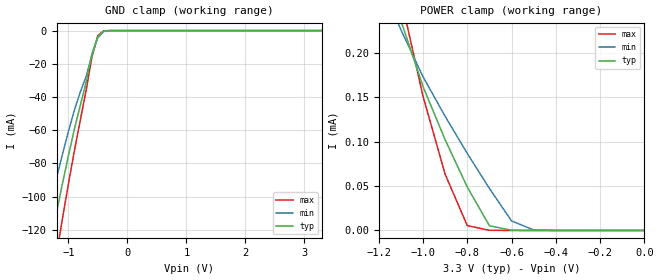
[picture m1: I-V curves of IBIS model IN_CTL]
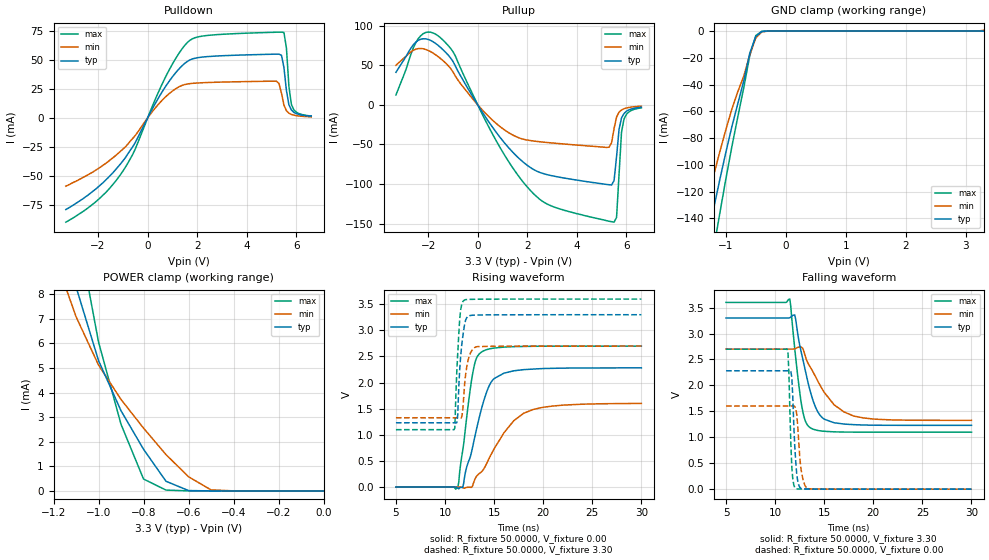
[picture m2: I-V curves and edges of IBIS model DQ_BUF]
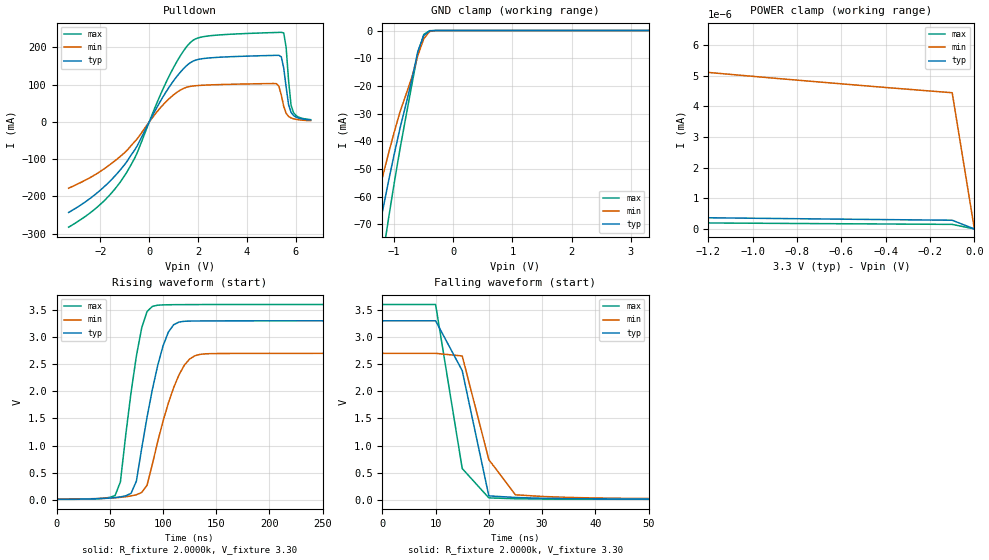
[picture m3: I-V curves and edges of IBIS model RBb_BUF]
| This IBIS file was created by s2ibis3 version 1.1
| North Carolina State University, ERL, 2006
[IBIS ver] 3.2
[File name] s34ml02g2_d_i_33_r2.ibs
[File Rev] 2.0
|   Rev1.0 Initial release with measurement
|   (X8 Legacy/ONFI F32 98799A 41122)
|   Rev2.0 Update 0A for 0V
[Date] 7/23/2014
[Source] Spansion IBIS team
|   Email: dl.ibisteam@spansion.com
[Notes]  Generated IBIS models from SPICE simulations.
|   VIO=3.3V, Temperature Range: Industrial (-40oC to +90oC).
[Disclaimer] THE MODEL LIBRARIES ARE PROVIDED AS IS.
[Copyright] (C) COPYRIGHT 2014
| SPANSION LLC
| ALL RIGHTS RESERVED.
|   Component S34ML02G2 X8 LEGACY/ONFI F32 in VBT067 package
[Component]   S34ML02G2
[Manufacturer]   Spansion
[Package]
| variable   typ   min   max
R_pkg   139.8mOhm   83.414mOhm   221.06mOhm
L_pkg   4.331nH   2.162nH   7.708nH
C_pkg   0.8614pF   0.3971pF   1.325pF
[Pin]   signal_name   model_name   R_pin   L_pin   C_pin
A2   NC   NC
A3   NC   NC
A6   NC   NC
A7   NC   NC
A8   NC   NC
B1   NC   NC
B2   WP   IN_CTL   186.22m   5.30n   1.33p
B3   ALE   IN_CTL   183.76m   5.66n   1.15p
B4   VSS   GND
B5   CE   IN_CTL   193.1m   7.14n   1.17p
B6   WE   IN_CTL   211.06m   6.84n   1.27p
B7   R/B#   RBb_BUF   176.3m   6.17n   1.11p
B8   NC   NC
C1   NC   NC
C2   NC   NC
C3   RE   IN_CTL   185.42m   7.71n   0.81p
C4   CLE   IN_CTL   170.19m   4.4n   1.18p
C5   NC   NC
C6   NC   NC
C7   NC   NC
C8   NC   NC
D2   NC   NC
D3   NC   NC
D4   NC   NC
D5   NC   NC
D6   NC   NC
D7   NC   NC
E2   NC   NC
E3   NC   NC
E4   NC   NC
E5   NC   NC
E6   NC   NC
E7   NC   NC
F2   NC   NC
F3   NC   NC
F4   NC   NC
F5   NC   NC
F6   NC   NC
F7   NC   NC
G2   NC   NC
G3   IO0   DQ_BUF   109.68m   2.85n   0.779p
G4   NC   NC
G5   NC   NC
G6   NC   NC
G7   VCC   POWER
H1   NC   NC
H2   NC   NC
H3   IO1   DQ_BUF   96.013m   2.44n   0.655p
H4   NC   NC
H5   VCC   POWER
H6   IO5   DQ_BUF   105.71m   3.38n   0.558p
H7   IO7   DQ_BUF   110.99m   3.27n   0.735p
H8   NC   NC
J1   NC   NC
J2   VSS   GND
J3   IO2   DQ_BUF   89.696m   2.19n   0.633p
J4   IO3   DQ_BUF   93.132m   2.31n   0.589p
J5   IO4   DQ_BUF   102.28m   3.14n   0.574p
J6   IO6   DQ_BUF   83.414m   2.16n   0.392p
J7   VSS   GND
J8   NC   NC
K1   NC   NC
K2   NC   NC
K3   NC   NC
K6   NC   NC
K7   NC   NC
K8   NC   NC
| Models and submodels in the file (3): IN_CTL (Input), DQ_BUF (I/O), RBb_BUF (Open_drain)
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|   Model IN_CTL
[Model]   IN_CTL
Model_type   Input
Vinl =   1.3180
Vinh =   1.6630
C_comp   6.01pF   5.78pF   8.57pF
[Temperature Range]   25.0000   90.0000   -40.0000
[Voltage Range]   3.3000   2.7000   3.6000
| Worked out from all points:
|   GND clamp passes 1 mA (typ) near -0.42 V on its own axis
|   POWER clamp passes 1 mA (typ) near -1.80 V on its own axis
[GND_clamp]
| voltage   I(typ)   I(min)   I(max)
-3.3V     -563.9mA   -475.7mA   -665.6mA
-1.5V     -164.8mA   -133.7mA   -202.4mA
-1.4V     -145.8mA   -118.2mA   -179.3mA
-1.3V     -127.4mA   -103.2mA   -156.7mA
-1.2V     -109.5mA   -88.65mA   -134.7mA
-1.1V     -92.25mA   -74.51mA   -113.2mA
-900mV    -59.75mA   -48.15mA   -72.81mA
-700mV    -31.42mA   -27.84mA   -36.18mA
-600mV    -14.17mA   -14.52mA   -15.79mA
-500mV    -3.458mA   -4.259mA   -2.945mA
-400mV    -298.7uA   -518.7uA   -127.7uA
3.3V      292.5pA    10.73uA    139.6pA
[POWER_clamp]
| voltage   I(typ)   I(min)   I(max)
-3.3V     27.06A     13.23A     34.66A
-1.1V     236.4uA    226.1uA    262.5uA
-1V       162.2uA    173.2uA    151.3uA
-900mV    102.2uA    128.6uA    63.39uA
-800mV    48.96uA    86.76uA    5.425uA
-700mV    5.388uA    47.41uA    237.2nA
-600mV    176.5nA    10.73uA    6.564nA
-500mV    6.019nA    596nA      279.6pA
0V        0A         0A         0A
|   Model DQ_BUF
[Model]   DQ_BUF
Model_type   I/O
Polarity   Non-Inverting
Enable   Active-High
Vinl =   1.3180
Vinh =   1.6630
Vmeas =   1.65V
C_comp   2.54pF   2.48pF   2.73pF
[Temperature Range]   25.0000   90.0000   -40.0000
[Voltage Range]   3.3000   2.7000   3.6000
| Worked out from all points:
|   slope of the pulldown table from 0 to 0.495 V, typ, clamps not added: 25.6 ohm
|   slope of the pullup table from 0 to 0.495 V, typ, clamps not added: 20.9 ohm
|   GND clamp passes 1 mA (typ) near -0.42 V on its own axis
|   POWER clamp passes 1 mA (typ) near -0.75 V on its own axis
|   rising waveform, R_fixture 50.0000, V_fixture 0.00: 20-80 % time 1.92ns typ, 3.23ns min, 1.14ns max; typ from 0 V to 2.28 V
|   rising waveform, R_fixture 50.0000, V_fixture 3.30: 20-80 % time 465ps typ, 496ps min, 379ps max; typ from 1.23 V to 3.3 V
|   falling waveform, R_fixture 50.0000, V_fixture 3.30: 20-80 % time 1.58ns typ, 2.84ns min, 926ps max; typ from 3.3 V to 1.23 V
|   falling waveform, R_fixture 50.0000, V_fixture 0.00: 20-80 % time 346ps typ, 421ps min, 262ps max; typ from 2.28 V to 0 V
[GND_clamp]
| voltage   I(typ)   I(min)   I(max)
-3.3V     -1.531A    -857.2mA   -2.572A
-1.5V     -199.4mA   -161.9mA   -246.1mA
-1.4V     -176.3mA   -143.2mA   -217.6mA
-1.3V     -153.9mA   -125mA     -189.7mA
-1.2V     -132.2mA   -107.4mA   -162.6mA
-1.1V     -111.1mA   -90.32mA   -136.3mA
-900mV    -71.7mA    -58.5mA    -86.72mA
-700mV    -37.18mA   -33.68mA   -42.32mA
-600mV    -16.53mA   -17.62mA   -18.35mA
-500mV    -4.024mA   -5.179mA   -3.39mA
-400mV    -347uA     -622.1uA   -145.7uA
3.3V      401pA      577.4uA    196.4pA
[POWER_clamp]
| voltage   I(typ)   I(min)   I(max)
-3.3V     28.02A     13.67A     36.43A
-1.2V     12.2mA     9.687mA    16.8mA
-1.1V     8.304mA    7.091mA    10.97mA
-1V       5.304mA    5.122mA    6.06mA
-900mV    3.262mA    3.722mA    2.71mA
-800mV    1.696mA    2.556mA    484.6uA
-700mV    392.2uA    1.477mA    34.23uA
-600mV    15.16uA    577.4uA    1.674uA
-500mV    621.3nA    42.06uA    41.77nA
-400mV    23.44nA    2.247uA    920.4pA
0V        0A         0A         0A
[Pulldown]
| voltage   I(typ)   I(min)   I(max)
-3.3V     -78.9mA    -58.8mA    -89.8mA
-1.1V     -39.8mA    -28.88mA   -49mA
-500mV    -21.23mA   -15.18mA   -26.87mA
900mV     32.53mA    21.5mA     42.55mA
1.8V      50.8mA     29.79mA    68.12mA
5.2V      54.94mA    31.61mA    73.89mA
5.4V      53.96mA    21.3mA     73.98mA
5.5V      43.4mA     11.1mA     73.57mA
5.6V      23.6mA     6.2mA      60.2mA
5.7V      11.3mA     4.1mA      27.2mA
5.8V      6.9mA      3mA        11.6mA
6.6V      1.6mA      900uA      1.8mA
[Pullup]
| voltage   I(typ)   I(min)   I(max)
-3.3V     41mA       49.8mA     12.4mA
-2.4V     81.3mA     70.88mA    83.4mA
-1.7V     77.37mA    63.08mA    89.09mA
-1V       54.74mA    41.53mA    67.09mA
700mV     -32.73mA   -22.28mA   -42.8mA
2.2V      -80.59mA   -45.42mA   -110.5mA
5.3V      -100.8mA   -53.4mA    -146.8mA
5.5V      -95.4mA    -29.8mA    -148mA
5.6V      -65.2mA    -15.4mA    -141.9mA
5.8V      -16.5mA    -6.5mA     -34.4mA
5.9V      -11mA      -4.9mA     -18mA
6.6V      -3.1mA     -1.7mA     -3.9mA
[Ramp]
| variable   typ   min   max
dV/dt_r   2.2818/1.922e-09   1.6009/3.212e-09   2.6978/1.138e-09
dV/dt_f   2.0696/1.584e-09   1.3732/2.799e-09   2.5018/9.242e-10
R_load = 50.0000
[Rising Waveform]
R_fixture = 50.0000
V_fixture = 0.00
| time   V(typ)   V(min)   V(max)
5ns       0V         0V         0V
11.3ns    -21.43mV   33.17uV    -13.34mV
11.8ns    -8.737mV   -10.81mV   695.5mV
12.9ns    842.8mV    76.14mV    2.255V
13.3ns    1.182V     224.4mV    2.504V
13.9ns    1.621V     332.1mV    2.606V
15ns      2.077V     731mV      2.662V
18ns      2.248V     1.411V     2.692V
22ns      2.277V     1.568V     2.697V
30ns      2.282V     1.601V     2.698V
[Rising Waveform]
R_fixture = 50.0000
V_fixture = 3.30
V_fixture_min = 2.70
V_fixture_max = 3.60
| time   V(typ)   V(min)   V(max)
5ns       1.23V      1.327V     1.098V
11ns      1.23V      1.327V     1.126V
11.2ns    1.231V     1.327V     2.214V
11.3ns    1.394V     1.327V     2.572V
11.5ns    2.262V     1.322V     3.228V
11.8ns    2.866V     1.452V     3.546V
12ns      3.122V     1.977V     3.582V
12.5ns    3.283V     2.523V     3.594V
13.2ns    3.294V     2.685V     3.596V
30ns      3.3V       2.7V       3.6V
[Falling Waveform]
R_fixture = 50.0000
V_fixture = 3.30
V_fixture_min = 2.70
V_fixture_max = 3.60
| time   V(typ)   V(min)   V(max)
5ns       3.3V       2.7V       3.6V
11.5ns    3.305V     2.7V       3.664V
12ns      3.357V     2.706V     2.703V
12.7ns    2.606V     2.733V     1.617V
13.1ns    2.264V     2.547V     1.304V
13.7ns    1.805V     2.313V     1.171V
14.3ns    1.507V     2.101V     1.134V
15ns      1.35V      1.866V     1.115V
18ns      1.244V     1.41V      1.1V
30ns      1.23V      1.327V     1.098V
[Falling Waveform]
R_fixture = 50.0000
V_fixture = 0.00
| time   V(typ)   V(min)   V(max)
5ns       2.282V     1.603V     2.698V
11.3ns    2.282V     1.603V     2.671V
11.4ns    2.283V     1.603V     2.243V
11.6ns    2.265V     1.603V     880.5mV
11.7ns    2.158V     1.605V     421.3mV
12.1ns    524.6mV    1.55V      10mV
12.3ns    158.3mV    1.219V     4.58mV
12.6ns    17.13mV    438.4mV    2.749mV
13.3ns    2.691mV    14.67mV    1.287mV
30ns      0V         641.2nV    0V
|   Model RBb_BUF
[Model]   RBb_BUF
Model_type   Open_drain
Polarity   Non-Inverting
Enable   Active-High
Vmeas =   1.65V
Rref =  2.0000k
Vref =  3.3000
C_comp   6.45pF   6.07pF   9.98pF
[Temperature Range]   25.0000   90.0000   -40.0000
[Voltage Range]   3.3000   2.7000   3.6000
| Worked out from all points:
|   slope of the pulldown table from 0 to 0.495 V, typ, clamps not added: 8.28 ohm
|   GND clamp passes 1 mA (typ) near -0.45 V on its own axis
|   POWER clamp passes 1 mA (typ) near -2.01 V on its own axis
|   rising waveform, R_fixture 2.0000k, V_fixture 3.30: 20-80 % time 19.6ns typ, 23.4ns min, 14.9ns max; typ from 0.013 V to 3.3 V
|   falling waveform, R_fixture 2.0000k, V_fixture 3.30: 20-80 % time 5.13ns typ, 5.19ns min, 3.56ns max; typ from 3.3 V to 0.013 V
[GND_clamp]
| voltage   I(typ)   I(min)   I(max)
-3.3V     -366.9mA   -293.6mA   -456.9mA
-1.5V     -100.2mA   -80.18mA   -128.1mA
-1.4V     -88.25mA   -70.88mA   -112.4mA
-1.3V     -76.7mA    -61.86mA   -97.26mA
-1.2V     -65.58mA   -53.15mA   -82.61mA
-1.1V     -54.91mA   -44.75mA   -68.56mA
-900mV    -35.17mA   -29.31mA   -42.57mA
-700mV    -17.63mA   -16.78mA   -19.44mA
-600mV    -7.539mA   -8.992mA   -8.14mA
-500mV    -1.807mA   -2.957mA   -1.425mA
-400mV    -154.4uA   -343.9uA   -57.58uA
3.3V      277.7pA    4.735nA    133.2pA
[POWER_clamp]
| voltage   I(typ)   I(min)   I(max)
-3.3V     1.67A      608.7mA    3.4A
-2.1V     9.427mA    14nA       295.6mA
-2V       303.3uA    6.064nA    92.6mA
-1.9V     7.905uA    5.601nA    4.048mA
-1.8V     205nA      5.511nA    40.63uA
-1.7V     5.702nA    5.44nA     380.1nA
-1.6V     535.8pA    5.372nA    3.762nA
-1.5V     393.7pA    5.304nA    242pA
-1.4V     381.8pA    5.237nA    204.8pA
-100mV    284.5pA    4.444nA    149.5pA
0V        0A         0A         0A
[Pulldown]
| voltage   I(typ)   I(min)   I(max)
-3.3V     -243.1mA   -178.1mA   -282.5mA
-1.1V     -122.1mA   -87.85mA   -153.2mA
-500mV    -65.05mA   -46.01mA   -83.83mA
900mV     101.5mA    67.22mA    134.1mA
1.9V      165.6mA    96.88mA    222.7mA
5.2V      178.4mA    102.3mA    239.7mA
5.4V      174.4mA    72.03mA    240.1mA
5.5V      144.4mA    41.6mA     238.5mA
5.6V      92.7mA     22.6mA     198.7mA
5.8V      25.3mA     10.5mA     44.7mA
6V        12.8mA     6.7mA      17.2mA
6.6V      5.1mA      3.2mA      5.9mA
[Ramp]
| variable   typ   min   max
dV/dt_r   2.8332/2.379e-08   2.1685/3.033e-08   3.2023/1.743e-08
dV/dt_f   2.8261/1.790e-08   2.1396/3.173e-08   3.2012/1.043e-08
R_load = 50.0000
[Rising Waveform]
R_fixture = 2.0000k
V_fixture = 3.30
V_fixture_min = 2.70
V_fixture_max = 3.60
| time   V(typ)   V(min)   V(max)
0s        12.68mV    14.86mV    10.59mV
55ns      42.37mV    39.93mV    80.39mV
60ns      55.15mV    47.84mV    332.1mV
75ns      346.4mV    94.68mV    2.651V
80ns      949.9mV    137.4mV    3.171V
90ns      2.033V     656.3mV    3.565V
105ns     3.09V      1.781V     3.595V
120ns     3.291V     2.48V      3.598V
135ns     3.297V     2.682V     3.599V
495ns     3.3V       2.7V       3.6V
[Falling Waveform]
R_fixture = 2.0000k
V_fixture = 3.30
V_fixture_min = 2.70
V_fixture_max = 3.60
| time   V(typ)   V(min)   V(max)
0s        3.3V       2.7V       3.6V
10ns      3.3V       2.7V       3.6V
15ns      2.381V     2.652V     577.9mV
20ns      74.22mV    741.6mV    37.37mV
25ns      44.85mV    94.16mV    21.35mV
30ns      29.93mV    63.6mV     15.81mV
40ns      19.68mV    35.16mV    12.67mV
105ns     13.24mV    16.77mV    10.69mV
495ns     12.68mV    14.86mV    10.59mV
